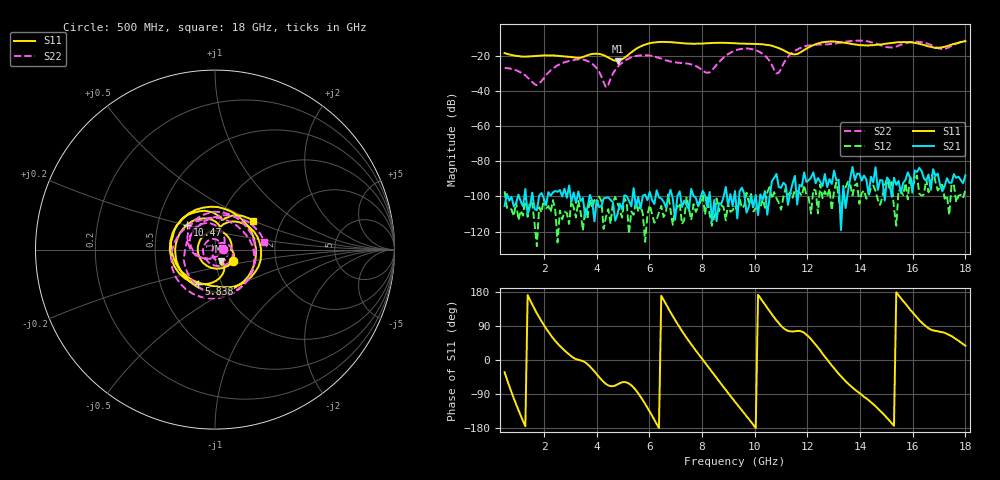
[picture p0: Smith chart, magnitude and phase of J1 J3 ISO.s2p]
!Agilent Technologies,N5230A,MY45001360,A.07.50.67
!Agilent N5230A: A.07.50.67
!Date: Tuesday, April 16, 2024 17:36:20
!Correction: S11(Full 2 Port(1,2))
!S21(Full 2 Port(1,2))
!S12(Full 2 Port(1,2))
!S22(Full 2 Port(1,2))
!S2P File: Measurements: S11, S21, S12, S22:
# Hz S  dB  R 50
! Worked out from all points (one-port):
!   201 points, 500 MHz to 18 GHz, reference 50 ohm
!   lowest |S11| = -22.7 dB at 4.787 GHz (marker M1), VSWR 1.16, Z = 52.8 - j6.99 ohm
!   |S11| at or under -10 dB: start of sweep to end of sweep
!   S11 on the Smith chart (normalised r, x): 500 MHz: 1.22, -0.16; 5.838 GHz: 0.78, -0.31; 10.47 GHz: 0.71, +0.21; 18 GHz: 1.43, +0.50
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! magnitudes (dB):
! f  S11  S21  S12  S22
! 500 MHz  -18.3  -105.4  -97.0  -26.9
! 1.025 GHz  -20.0  -98.9  -113.5  -28.6
! 1.725 GHz  -19.9  -107.9  -128.3  -36.6
! 2.513 GHz  -19.8  -97.3  -126.2  -25.2
! 3.475 GHz  -20.5  -101.0  -119.4  -22.0
! 4 GHz  -18.6  -102.1  -105.1  -27.0
! 4.35 GHz  -20.1  -100.8  -111.5  -37.9
! 4.787 GHz  -22.7  -110.1  -103.9  -26.3
! 5.838 GHz  -13.4  -98.9  -125.9  -19.5
! 6.362 GHz  -12.0  -100.6  -109.3  -21.0
! 8.2 GHz  -12.7  -106.1  -100.6  -29.5
! 9.25 GHz  -12.7  -96.9  -105.1  -16.9
! 9.95 GHz  -13.1  -106.1  -108.5  -16.2
! 10.47 GHz  -13.6  -110.4  -97.7  -21.2
! 10.82 GHz  -14.9  -87.2  -101.1  -29.9
! 11.44 GHz  -19.0  -92.5  -100.7  -17.9
! 12.22 GHz  -13.8  -86.3  -96.0  -13.7
! 14.06 GHz  -13.8  -91.0  -98.0  -11.2
! 15.11 GHz  -12.7  -91.0  -95.1  -15.0
! 16.16 GHz  -12.8  -86.0  -88.1  -11.8
! 17.21 GHz  -14.6  -94.1  -101.3  -16.0
! 18 GHz  -11.5  -87.9  -96.2  -11.1
